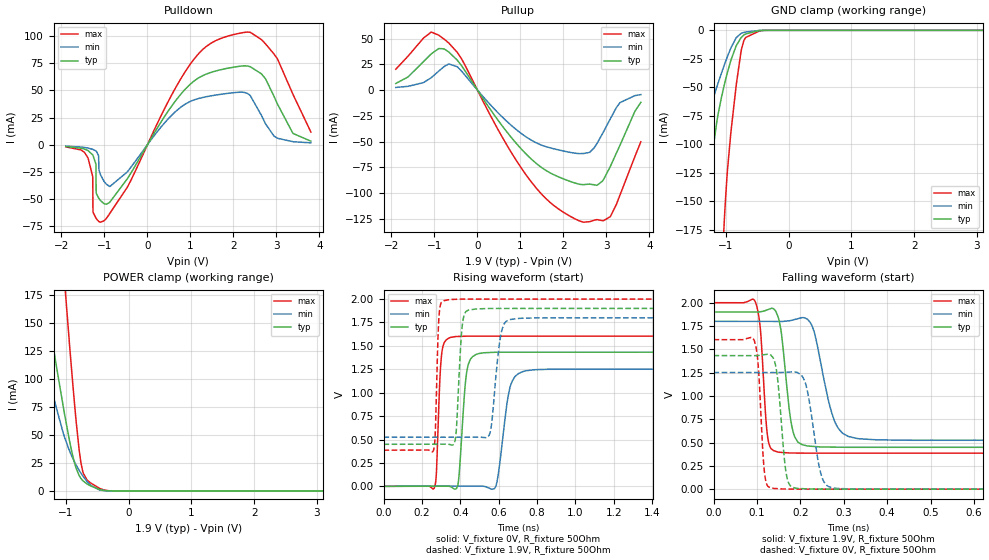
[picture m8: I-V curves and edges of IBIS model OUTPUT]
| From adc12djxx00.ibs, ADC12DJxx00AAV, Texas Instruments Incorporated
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|   Model OUTPUT
[Model]   OUTPUT
Model_type   3-state
Polarity   Non-Inverting
Vmeas = 0.95
Vref = 1.9
Cref = 15pF
Rref = 50
|   (nom PVT)   (slow PVT)   (fast PVT)
|   typ   min   max
C_comp   0.807p   0.780p   0.910p
|C_comp (High state)   0.807p   0.780p   0.910p
|C_comp (Low state)   0.869p   0.766p   0.951p
|C_comp (OFF state)   0.837p   0.7690p   0.917p
[Voltage Range]   1.9   1.8   2
[Temperature Range]   27   125   -40
[Pullup Reference]   1.9   1.8   2
[Pulldown Reference]   0   0   0
[Power Clamp Reference]   1.9   1.8   2
[GND Clamp Reference]   0   0   0
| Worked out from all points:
|   slope of the pulldown table from 0 to 0.285 V, typ, clamps not added: 15 ohm
|   slope of the pullup table from 0 to 0.285 V, typ, clamps not added: 15.9 ohm
|   GND clamp passes 1 mA (typ) near -0.53 V on its own axis
|   POWER clamp passes 1 mA (typ) near -0.45 V on its own axis
|   falling waveform, V_fixture 1.9V, R_fixture 50Ohm: 20-80 % time 20ps typ, 36.2ps min, 12.8ps max; typ from 1.9 V to 0.449 V
|   rising waveform, V_fixture 0V, R_fixture 50Ohm: 20-80 % time 29.2ps typ, 47.2ps min, 18.6ps max; typ from 0 V to 1.43 V
|   rising waveform, V_fixture 1.9V, R_fixture 50Ohm: 20-80 % time 22.3ps typ, 36.5ps min, 13.6ps max; typ from 0.449 V to 1.9 V
|   falling waveform, V_fixture 0V, R_fixture 50Ohm: 20-80 % time 15.7ps typ, 24.6ps min, 11.1ps max; typ from 1.43 V to 0 V
[Pulldown]
|   Voltage   I(typ)   I(min)   I(max)
-1.9V     -1.671mA   -1.357mA   -2mA
-1.387V   -5.34mA    -3.104mA   -11.92mA
-1.273V   -9.514mA   -4.318mA   -29.44mA
-1.267V   -9.868mA   -4.405mA   -62.15mA
-1.199V   -17.95mA   -5.864mA   -67.63mA
-1.193V   -44.56mA   -6.042mA   -67.98mA
-1.011V   -54.44mA   -33.89mA   -70.26mA
1.047V    57.51mA    40.73mA    77.01mA
2.324V    72.51mA    47.22mA    103.8mA
2.945V    44.38mA    7.798mA    83.46mA
3.384V    10.35mA    2.729mA    46.38mA
3.8V      3.24mA     1.677mA    11.65mA
[GND Clamp]
|   Voltage   I(typ)   I(min)   I(max)
-1.9V     -468.1mA   -241.3mA   -1.492A
-1.535V   -268.5mA   -129.4mA   -909.9mA
-1.37V    -181.5mA   -89.41mA   -651.1mA
-1.153V   -82.39mA   -50.77mA   -326.2mA
-1.028V   -47.9mA    -30.43mA   -167mA
-976.6mV  -36.65mA   -22.78mA   -122.3mA
-925.3mV  -26.74mA   -15.79mA   -90.99mA
-834.1mV  -13.2mA    -6.251mA   -46.61mA
-760mV    -6.433mA   -2.699mA   -18.22mA
-685.9mV  -3.159mA   -1.485mA   -6.252mA
-406.6mV  -42.65uA   -30.48uA   -129.5uA
3.8V      0A         0A         0A
[Pullup]
|   Voltage   I(typ)   I(min)   I(max)
-1.9V     6.464mA    2.606mA    20.35mA
-1.079V   35.06mA    11.94mA    56.37mA
-742.9mV  39.24mA    23.78mA    48.49mA
-469.3mV  29.1mA     22.74mA    36.69mA
568.1mV   -34.35mA   -25.81mA   -45.06mA
1.206V    -65.24mA   -47.51mA   -86.75mA
1.765V    -82.04mA   -56.95mA   -111.8mA
2.455V    -91.9mA    -61.67mA   -128.3mA
2.78V     -92.56mA   -51.9mA    -125.9mA
3.093V    -73.96mA   -27.65mA   -122.8mA
3.316V    -53.53mA   -12.14mA   -101.9mA
3.8V      -11.83mA   -4.362mA   -50.18mA
[POWER Clamp]
|   Voltage   I(typ)   I(min)   I(max)
-1.9V     378.9mA    258.1mA    917.9mA
-1.472V   223.6mA    150mA      553mA
-1.319V   168.8mA    112.3mA    423.7mA
-1.153V   111.4mA    73.96mA    287.8mA
-1.022V   68.14mA    47.7mA     186.2mA
-948.1mV  45.79mA    36.27mA    133.3mA
-874mV    26.95mA    26.97mA    83.62mA
-788.5mV  13.49mA    18.19mA    35.51mA
-725.8mV  8.786mA    12.85mA    15.84mA
-611.8mV  4.547mA    5.207mA    7.245mA
-286.9mV  39.79uA    36.14uA    80.39uA
3.8V      0A         0A         0A
[Ramp]
R_load = 50
|   typ   min   max
dV/dt_r   0.859575/2.91839e-11   0.750624/4.67569e-11   0.962384/1.85514e-11
dV/dt_f   0.87071/1.99793e-11   0.76565/3.60101e-11   0.968465/1.27389e-11
[Falling Waveform]
V_fixture = 1.9V
V_fixture_min = 1.8V
V_fixture_max = 2V
R_fixture = 50Ohm
C_fixture = 0F
|   Time   V(typ)   V(min)   V(max)
0s        1.9V       1.8V       2V
96.44ps   1.899V     1.799V     2.008V
108.4ps   1.903V     1.799V     1.693V
125ps     1.925V     1.799V     551.6mV
148.5ps   1.852V     1.799V     397.9mV
181.7ps   646.9mV    1.813V     387.9mV
214.7ps   465mV      1.827V     386.4mV
280.4ps   450.7mV    714.2mV    386mV
330.7ps   449.1mV    543.8mV    386mV
1.8ns     448.8mV    523.9mV    385.9mV
[Rising Waveform]
V_fixture = 0V
V_fixture_min = 0V
V_fixture_max = 0V
R_fixture = 50Ohm
C_fixture = 0F
|   Time   V(typ)   V(min)   V(max)
0s        108.1nV    605.2nV    903.3nV
265.5ps   1.442mV    879.5uV    -13.83mV
301.5ps   1.637mV    998.5uV    1.381V
342.3ps   276.4uV    1.134mV    1.585V
387.9ps   18.61mV    1.285mV    1.601V
433.2ps   1.213V     1.435mV    1.604V
481.9ps   1.408V     1.596mV    1.604V
585.7ps   1.432V     427.9uV    1.604V
724.3ps   1.432V     1.224V     1.604V
1.8ns     1.433V     1.251V     1.604V
[Rising Waveform]
V_fixture = 1.9V
V_fixture_min = 1.8V
V_fixture_max = 2V
R_fixture = 50Ohm
C_fixture = 0F
|   Time   V(typ)   V(min)   V(max)
0s        448.8mV    523.9mV    385.9mV
260.3ps   449.8mV    524.2mV    382.1mV
289.1ps   449.9mV    524.3mV    1.808V
311.1ps   450mV      524.3mV    1.98V
373.9ps   496.8mV    524.4mV    1.997V
409.2ps   1.69V      524.4mV    2V
440.1ps   1.88V      524.4mV    2V
551.1ps   1.899V     547.5mV    2V
653.3ps   1.9V       1.778V     2V
1.8ns     1.9V       1.8V       2V
[Falling Waveform]
|Gnd
V_fixture = 0V
V_fixture_min = 0V
V_fixture_max = 0V
R_fixture = 50Ohm
C_fixture = 0F
|   Time   V(typ)   V(min)   V(max)
0s        1.433V     1.251V     1.604V
93.94ps   1.432V     1.251V     1.595V
102.9ps   1.434V     1.251V     1.331V
118.3ps   1.443V     1.251V     147.4mV
135ps     1.423V     1.25V      10.96mV
167.6ps   164.1mV    1.254V     1.595mV
189.3ps   10.91mV    1.255V     762.7uV
249.3ps   1.153mV    135.3mV    102.6uV
275.8ps   237.6uV    12.42mV    100.8uV
1.8ns     106.7nV    620.6nV    921.6nV
